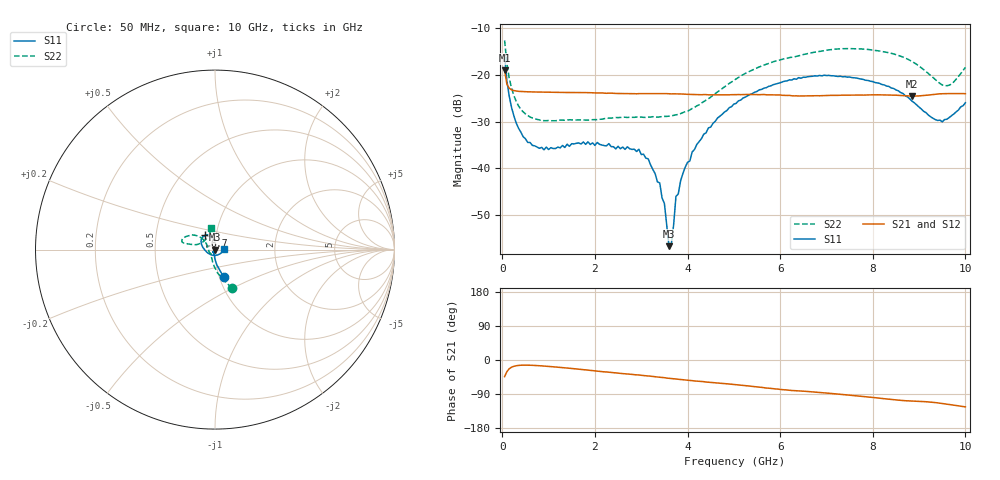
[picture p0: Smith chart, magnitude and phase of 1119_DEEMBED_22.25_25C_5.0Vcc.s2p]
!Hittite Microwave Corp.
!Digital Attenuator/PhaseShifter Rev 1.4.0
!Filename: C:\DATA\DATA\1119_DEEMBED_22.25_25C_5.0Vcc.s2p
!VNA ID: Agilent Technologies,N5224A,MY51441122,A.10.45.03
!Device type:
!2 Port Calibration.
!Temp(C): 25
!Lot Number:
!Serial Number:
!Operator:
!Misc:
!Attenuator:  22.250
# GHZ S DB R 50.0
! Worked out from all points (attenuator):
!   200 points, 50 MHz to 10 GHz, reference 50 ohm
!   highest |S21| = -19.03 dB at 50 MHz (marker M1); lowest = -24.6 dB at 8.85 GHz (marker M2)
!   lowest |S11| = -56.8 dB at 3.6 GHz (marker M3), VSWR 1.00, Z = 49.9 + j0.00228 ohm
!   |S11| at or under -10 dB: start of sweep to end of sweep
!   |S22| runs from -29.8 to -12.6 dB; largest |S21 - S12| = 0.00018
!   S11 on the Smith chart (normalised r, x): 50 MHz: 1.05, -0.33; 6.7 GHz: 0.88, +0.14; 10 GHz: 1.11, +0.01
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0.05  -15.89 -72.5  -19.03 -43.9  -19.04 -43.9  -12.60 -66.6
0.1  -21.34 -83.2  -22.02 -30.6  -22.02 -30.6  -17.56 -83.5
0.2  -26.99 -92.3  -23.20 -18.9  -23.20 -18.9  -22.84 -100.2
0.35  -31.42 -99.5  -23.52 -14.3  -23.51 -14.3  -26.63 -114.1
0.55  -34.49 -108.5  -23.62 -13.6  -23.61 -13.6  -28.71 -125.8
0.9  -36.06 -116.6  -23.69 -15.9  -23.69 -16.0  -29.81 -135.1
1.75  -34.39 -125.2  -23.79 -25.4  -23.79 -25.5  -29.67 -139.7
2.95  -35.94 -111.9  -24.01 -39.6  -24.01 -39.6  -29.06 -158.7
3.4  -43.17 -123.9  -24.01 -45.4  -24.01 -45.4  -28.99 -172.1
3.5  -47.57 -134.8  -23.99 -46.7  -24.00 -46.8  -28.90 -175.7
3.6  -56.75 179.1  -24.05 -48.3  -24.05 -48.3  -28.85 -179.7
3.65  -56.32 124.7  -24.07 -48.7  -24.08 -48.8  -28.79 178.8
3.75  -46.07 105.3  -24.06 -50.2  -24.07 -50.2  -28.56 174.7
4.1  -36.53 86.8  -24.16 -54.5  -24.16 -54.5  -27.21 159.6
4.45  -31.37 84.5  -24.27 -58.6  -24.29 -58.7  -25.09 147.4
5.05  -26.10 95.4  -24.23 -65.2  -24.25 -65.2  -20.85 139.5
5.85  -22.10 110.5  -24.27 -75.7  -24.28 -75.8  -17.17 144.6
6.7  -20.28 125.4  -24.45 -84.2  -24.46 -84.2  -15.19 154.5
8.35  -22.48 163.8  -24.32 -103.4  -24.32 -103.4  -15.24 168.2
8.85  -25.64 -172.1  -24.55 -108.3  -24.55 -108.3  -17.14 167.8
9.55  -29.58 -67.7  -24.01 -115.8  -24.02 -115.8  -22.29 138.9
10  -25.97 3.6  -24.03 -123.7  -24.04 -123.7  -18.39 99.6
